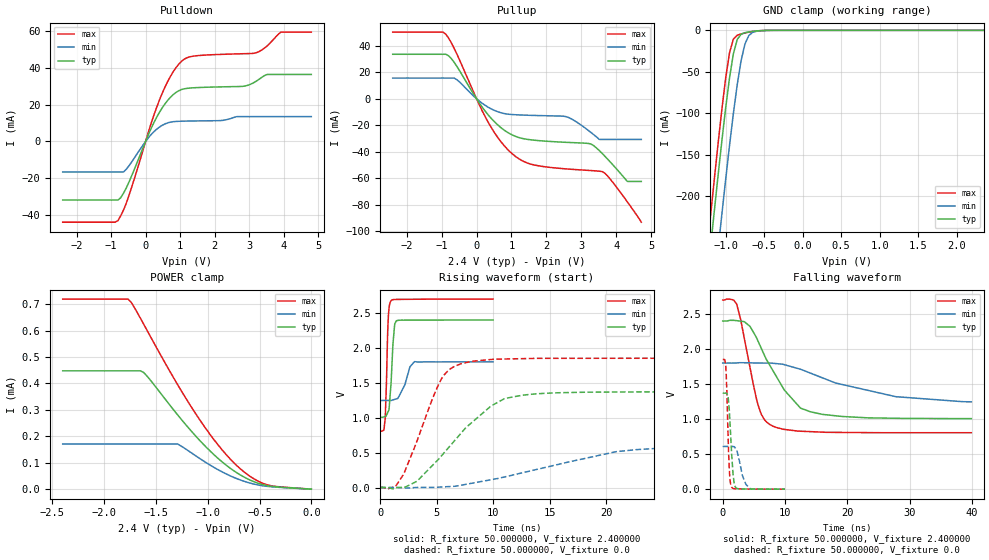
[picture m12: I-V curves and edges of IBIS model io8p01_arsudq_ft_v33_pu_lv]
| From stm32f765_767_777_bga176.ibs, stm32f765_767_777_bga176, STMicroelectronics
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|   Model io8p01_arsudq_ft_v33_pu_lv
[Model]  io8p01_arsudq_ft_v33_pu_lv
Model_type I/O
Polarity   Non-Inverting
Enable   Active-Low
Vinl =   0.720000V
Vinh =   1.680000V
Vmeas =  1.200000V
Cref =   50.000000pF
Rref =   100.000000M
Vref =   0.0V
C_comp   2.238700pF   2.180600pF   2.332300pF
[Temperature Range]   25.000000   0.125000k   -40.000000
[Pullup Reference]   2.400000V   1.800000V   2.700000V
[Pulldown Reference]   0.0V   0.0V   0.0V
[POWER Clamp Reference]   2.400000V   1.800000V   2.700000V
[GND Clamp Reference]   0.0V   0.0V   0.0V
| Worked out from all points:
|   slope of the pulldown table from 0 to 0.36 V, typ, clamps not added: 25 ohm
|   slope of the pullup table from 0 to 0.36 V, typ, clamps not added: 27.7 ohm
|   GND clamp passes 1 mA (typ) near -0.62 V on its own axis
|   rising waveform, R_fixture 50.000000, V_fixture 2.400000: 20-80 % time 302ps typ, 741ps min, 198ps max; typ from 1.01 V to 2.4 V
|   rising waveform, R_fixture 50.000000, V_fixture 0.0: 20-80 % time 4.92ns typ, 9.98ns min, 2.66ns max; typ from 0.001 V to 1.37 V
|   falling waveform, R_fixture 50.000000, V_fixture 2.400000: 20-80 % time 5.56ns typ, 12.8ns min, 2.64ns max; typ from 2.4 V to 1.01 V
|   falling waveform, R_fixture 50.000000, V_fixture 0.0: 20-80 % time 535ps typ, 1.03ns min, 387ps max; typ from 1.37 V to 0.001 V
[Pulldown]
|Voltage   I(typ)   I(min)   I(max)
-2.4V     -31.73mA   -16.51mA   -43.74mA
-800mV    -31.73mA   -16.51mA   -42.87mA
-480mV    -21.98mA   -13.17mA   -29.21mA
80mV      3.63mA     1.966mA    5.014mA
480mV     18.16mA    8.738mA    26.02mA
800mV     25.38mA    10.72mA    37.77mA
1.12V     28.53mA    11.02mA    44.6mA
2.8V      29.84mA    13.45mA    47.53mA
3.2V      32.59mA    13.45mA    48.03mA
3.52V     36.3mA     13.45mA    51.74mA
3.92V     36.3mA     13.45mA    59.27mA
4.8V      36.3mA     13.45mA    59.27mA
[Pullup]
|Voltage   I(typ)   I(min)   I(max)
-2.4V     33.49mA    15.55mA    50.22mA
-960mV    33.49mA    15.55mA    50.22mA
-800mV    32.39mA    15.55mA    45.71mA
-560mV    24.27mA    14.29mA    33.52mA
320mV     -11.75mA   -6.207mA   -17.08mA
960mV     -26.47mA   -11.82mA   -40.02mA
1.52V     -30.88mA   -12.51mA   -49.05mA
2.56V     -32.88mA   -13.48mA   -52.9mA
3.28V     -34.18mA   -25.5mA    -54.17mA
3.6V      -41.3mA    -30.74mA   -54.97mA
4.32V     -62.38mA   -30.74mA   -77.8mA
4.72V     -62.38mA   -30.74mA   -93.1mA
[GND_clamp]
|Voltage   I(typ)   I(min)   I(max)
-2.4V     -1.424A    -1.508A    -1.394A
-1.25V    -311.2mA   -401.9mA   -273.3mA
-1.2V     -265.4mA   -356.1mA   -227.2mA
-1.15V    -220.4mA   -310.8mA   -181.9mA
-1.1V     -176.3mA   -266.2mA   -137.9mA
-1.05V    -133.8mA   -222.5mA   -95.87mA
-950mV    -57.3mA    -138.9mA   -26.98mA
-900mV    -28.27mA   -100.4mA   -10.59mA
-850mV    -11.01mA   -65.54mA   -5.958mA
-750mV    -2.834mA   -16.5mA    -3.178mA
-600mV    -750uA     -1.164mA   -738.3uA
2.35V     0A         0A         0A
[POWER_clamp]
|Voltage   I(typ)   I(min)   I(max)
-2.4V     447.7uA    170.8uA    719.3uA
-1.77V    447.7uA    170.8uA    719.3uA
-1.74V    447.7uA    170.8uA    707.6uA
-1.65V    447.7uA    170.8uA    647uA
-1.62V    442uA      170.8uA    625.5uA
-1.29V    280.9uA    170.8uA    395.1uA
-1.02V    161uA      101.5uA    230.1uA
-780mV    78.34uA    49.93uA    112.9uA
-600mV    36.03uA    23.94uA    50.74uA
-450mV    15.19uA    11.76uA    19.45uA
-330mV    8.429uA    7.427uA    9.749uA
0V        0A         0A         0A
[Ramp]
| variable   typ   min   max
dV/dt_r  0.82243/4.91558n   0.36486/10.00248n   1.11071/2.65663n
dV/dt_f  0.83646/5.56816n   0.32208/12.85477n   1.13666/2.64005n
R_load = 50.000000
[Rising Waveform]
R_fixture= 50.000000
V_fixture= 2.400000
V_fixture_min= 1.800000
V_fixture_max= 2.700000
|time   V(typ)   V(min)   V(max)
0s        1.007V     1.247V     806mV
320.3ps   1.012V     1.247V     824.2mV
440.4ps   1.017V     1.247V     1V
720.7ps   1.096V     1.247V     2.465V
961ps     1.517V     1.247V     2.676V
1.121ns   2.058V     1.255V     2.691V
1.281ns   2.343V     1.263V     2.694V
1.421ns   2.389V     1.27V      2.695V
3.023ns   2.398V     1.804V     2.697V
9.97ns    2.4V       1.8V       2.7V
[Rising Waveform]
R_fixture= 50.000000
V_fixture= 0.0
V_fixture_min= 0.0
V_fixture_max= 0.0
|time   V(typ)   V(min)   V(max)
0s        965.3uV    875.3uV    1.108mV
1.361ns   -5.94mV    468.9uV    21.5mV
2.002ns   5.193mV    -4.114mV   175.2mV
3.283ns   96.41mV    1.385mV    682.9mV
5.365ns   445.6mV    7.61mV     1.544V
7.207ns   790.5mV    35.15mV    1.776V
9.85ns    1.173V     113.6mV    1.835V
12.65ns   1.324V     214.7mV    1.847V
22.66ns   1.37V      543mV      1.852V
39.88ns   1.371V     610.3mV    1.852V
[Falling Waveform]
R_fixture= 50.000000
V_fixture= 2.400000
V_fixture_min= 1.800000
V_fixture_max= 2.700000
|time   V(typ)   V(min)   V(max)
0s        2.4V       1.8V       2.7V
2.242ns   2.405V     1.802V     2.641V
4.324ns   2.328V     1.804V     1.762V
5.606ns   2.125V     1.801V     1.223V
6.567ns   1.936V     1.8V       1.011V
7.768ns   1.736V     1.799V     912.6mV
9.93ns    1.41V      1.776V     853.2mV
14.09ns   1.105V     1.656V     821.6mV
27.79ns   1.012V     1.32V      806.1mV
39.88ns   1.007V     1.247V     806mV
[Falling Waveform]
R_fixture= 50.000000
V_fixture= 0.0
V_fixture_min= 0.0
V_fixture_max= 0.0
|time   V(typ)   V(min)   V(max)
0s        1.371V     610.3mV    1.852V
460.5ps   1.371V     610.1mV    1.79V
660.7ps   1.367V     610mV      1.398V
1.041ns   1.146V     609.7mV    312.8mV
1.421ns   522.6mV    610.6mV    32.79mV
1.802ns   108.9mV    607.4mV    9.203mV
2.202ns   15.81mV    566.1mV    6.112mV
3.143ns   4.025mV    200.2mV    4.098mV
4.364ns   3.08mV     9.294mV    2.6mV
9.97ns    965.3uV    875.3uV    1.108mV
